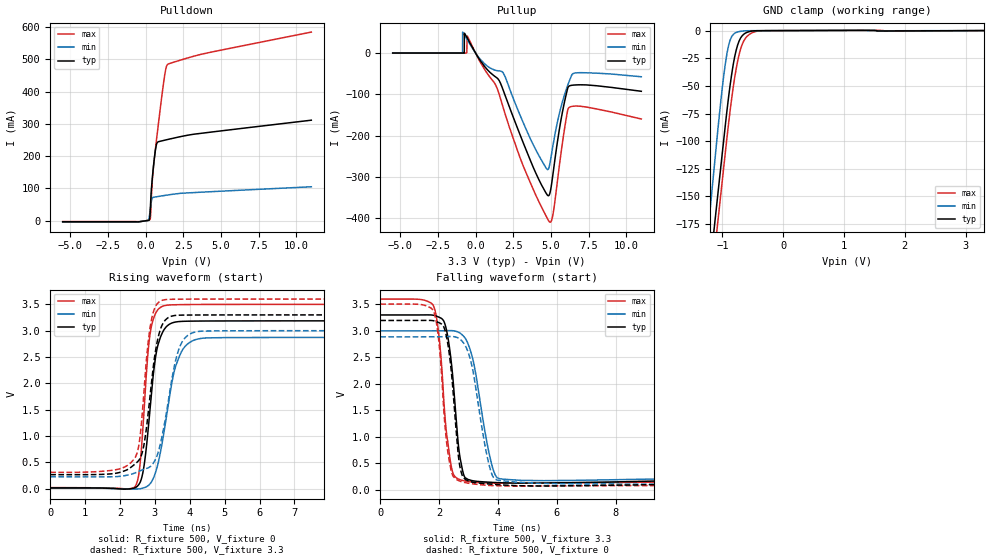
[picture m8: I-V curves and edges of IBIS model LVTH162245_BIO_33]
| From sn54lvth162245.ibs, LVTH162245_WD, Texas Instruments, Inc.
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[Model]   LVTH162245_BIO_33
Model_type  I/O
Vinl = 0.8
Vinh = 2.0
Enable   Active-Low
Vref =   0
Rref =   500
Cref =   50p
Vmeas =   1.5
| variable   typ   min   max
C_comp   10.0pF   NA   NA
| C_pullup   7.22pF   3.35pF   13.24pF
| C_pulldown   5.48pF   4.36pF   6.99pF
| C_tri-state   5.46pF   4.28pF   7.16pF
[Temperature Range]   40   -40   100
| Ambient temperature   25   -40   85
[Voltage range]   3.3   3   3.6
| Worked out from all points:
|   slope of the pulldown table from 0 to 0.495 V, typ, clamps not added: 3.18 ohm
|   slope of the pullup table from 0 to 0.495 V, typ, clamps not added: 18 ohm
|   GND clamp passes 1 mA (typ) near -0.56 V on its own axis
|   rising waveform, R_fixture 500, V_fixture 0: 20-80 % time 301ps typ, 458ps min, 228ps max; typ from 0.016 V to 3.19 V
|   falling waveform, R_fixture 500, V_fixture 3.3: 20-80 % time 301ps typ, 513ps min, 290ps max; typ from 3.3 V to 0.254 V
|   rising waveform, R_fixture 500, V_fixture 3.3: 20-80 % time 342ps typ, 467ps min, 267ps max; typ from 0.268 V to 3.3 V
|   falling waveform, R_fixture 500, V_fixture 0: 20-80 % time 306ps typ, 525ps min, 306ps max; typ from 3.2 V to 0.021 V
[GND Clamp]
| LVTH162245_BIO_33
|   Voltage   I(typ)   I(min)   I(max)
-5.5V     -2.999A    -3.125A    -3.027A
-1.26V    -242.6mA   -194.5mA   -268.5mA
-1.185V   -204mA     -151.9mA   -229mA
-1.075V   -147.8mA   -89.46mA   -172.6mA
-1V       -109.7mA   -50.57mA   -134.5mA
-925mV    -72.14mA   -20.58mA   -96.61mA
-875mV    -49.94mA   -8.862mA   -73.02mA
-800mV    -24.04mA   -2.465mA   -42.96mA
-725mV    -9.335mA   -904.5uA   -21.59mA
-650mV    -3.341mA   -325.1uA   -9.489mA
-415mV    -108.8uA   -86.1uA    -379.2uA
3.3V      31.16pA    26.13pA    -1.136uA
[Pulldown]
| LVTH162245_BIO_33
|   Voltage   I(typ)   I(min)   I(max)
-5.5V     -3.024mA   -4.072mA   -2.57mA
-530mV    -3.533mA   -3.753mA   -2.57mA
185mV     1.21mA     1.224mA    1.221mA
290mV     16.6mA     27.75mA    4.13mA
340mV     60.93mA    45.83mA    21.23mA
445mV     130.6mA    70.19mA    123mA
595mV     198.8mA    73.15mA    197.1mA
710mV     233.6mA    74.08mA    244.9mA
1.26V     249.5mA    78.33mA    448.2mA
1.37V     250.7mA    79.14mA    475.5mA
1.47V     251.7mA    79.86mA    484.5mA
11V       311.5mA    105.3mA    584.4mA
[Pullup]
| LVTH162245_BIO_33
|   Voltage   I(typ)   I(min)   I(max)
-5.5V     74.96uA    40.9uA     128.5uA
-865mV    62.1uA     38.1uA     109.8uA
-860mV    61.85uA    50.32mA    109.7uA
-755mV    43.26uA    44.66mA    101.1uA
-740mV    48.1mA     43.72mA    97.29uA
-600mV    39.62mA    35.02mA    94.91uA
-545mV    35.97mA    31.65mA    41.2mA
1.835V    -90.11mA   -48.14mA   -132.5mA
4.02V     -292.7mA   -236.1mA   -346.3mA
4.94V     -338.6mA   -266.6mA   -410mA
6.18V     -80.64mA   -71.64mA   -132.8mA
11V       -92.62mA   -57.42mA   -159.8mA
[Ramp]
| LVTH162245_BIO_33
| variable   typ   min   max
dV/dt_r   1.92/3.04E-10   1.73/4.72E-10   2.10/2.34E-10
dV/dt_f   1.90/3.23E-10   1.70/5.26E-10   2.08/3.19E-10
R_load = 500
[Rising Waveform]
| LVTH162245_BIO_33
R_fixture =   500
C_fixture =   0
L_fixture =   0
V_fixture =   0
V_fixture_min = 0
V_fixture_max = 0
|   Time   V(typ)   V(min)   V(max)
0s        16.34mV    10.25mV    21.6mV
2.435ns   20.33mV    -5.905mV   43.74mV
2.555ns   97.12mV    -1.818mV   358.9mV
2.665ns   343.2mV    14.34mV    1.244V
2.885ns   1.688V     115.3mV    3.032V
3.065ns   2.667V     416.4mV    3.38V
3.355ns   3.093V     1.471V     3.484V
3.765ns   3.176V     2.605V     3.494V
4.495ns   3.184V     2.863V     3.498V
50ns      3.188V     2.873V     3.5V
[Falling Waveform]
| LVTH162245_BIO_33
R_fixture =   500
C_fixture =   0
L_fixture =   0
V_fixture =   3.3
V_fixture_min = 3
V_fixture_max = 3.6
|   Time   V(typ)   V(min)   V(max)
0s        3.3V       3V         3.6V
1.79ns    3.296V     3.001V     3.493V
1.985ns   3.26V      3.001V     2.952V
2.155ns   3.188V     3.002V     1.716V
2.46ns    2.15V      3.003V     330.5mV
2.705ns   622.9mV    2.959V     192.3mV
3.03ns    187.7mV    2.683V     155mV
3.78ns    141.7mV    491.2mV    128.4mV
4.17ns    132mV      201.2mV    126mV
50ns      254.2mV    220.3mV    299.4mV
[Rising Waveform]
| LVTH162245_BIO_33
R_fixture =   500
C_fixture =   0
L_fixture =   0
V_fixture =   3.3
V_fixture_min = 3
V_fixture_max = 3.6
|   Time   V(typ)   V(min)   V(max)
0s        267.7mV    226.8mV    311.7mV
2.435ns   473mV      301.2mV    593.3mV
2.555ns   555.7mV    336.6mV    894.1mV
2.675ns   797.2mV    366.4mV    1.748V
2.9ns     2.001V     440.6mV    3.205V
3.095ns   2.88V      696mV      3.532V
3.335ns   3.224V     1.469V     3.592V
3.73ns    3.295V     2.721V     3.598V
4.38ns    3.298V     2.993V     3.6V
50ns      3.3V       3V         3.6V
[Falling Waveform]
| LVTH162245_BIO_33
R_fixture =   500
C_fixture =   0
L_fixture =   0
V_fixture =   0
V_fixture_min = 0
V_fixture_max = 0
|   Time   V(typ)   V(min)   V(max)
0s        3.196V     2.888V     3.505V
1.79ns    3.192V     2.889V     3.395V
1.98ns    3.158V     2.889V     2.849V
2.15ns    3.083V     2.889V     1.563V
2.405ns   2.277V     2.894V     369.7mV
2.71ns    423.1mV    2.841V     163.2mV
3.185ns   139.2mV    2.13V      110.2mV
3.81ns    105.4mV    268.4mV    80.35mV
4.645ns   78.2mV     144.5mV    71.69mV
50ns      20.7mV     12.81mV    24.44mV
